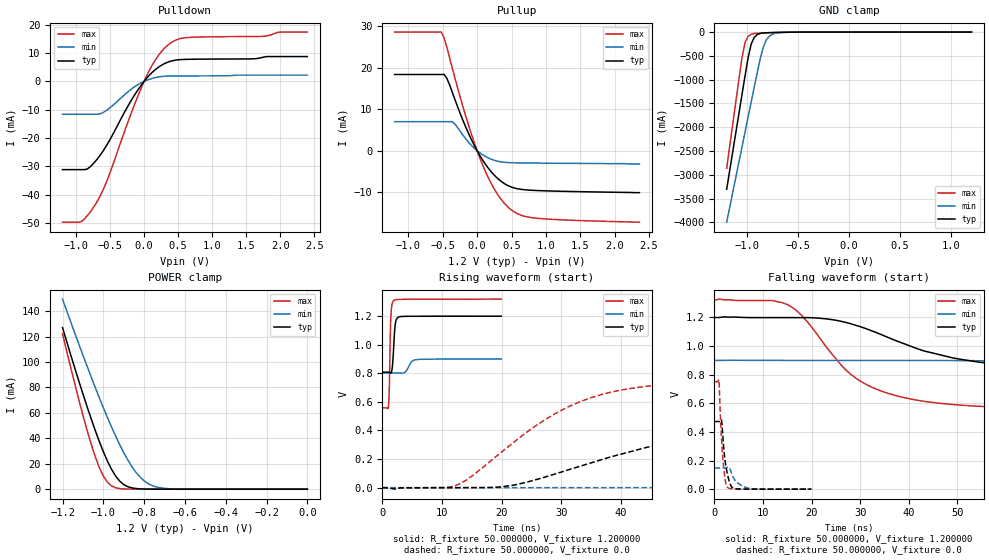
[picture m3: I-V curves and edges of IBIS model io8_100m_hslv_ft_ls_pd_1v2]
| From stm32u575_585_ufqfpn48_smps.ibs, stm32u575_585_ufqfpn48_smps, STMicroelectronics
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|   Model io8_100m_hslv_ft_ls_pd_1v2
[Model]  io8_100m_hslv_ft_ls_pd_1v2
Model_type I/O
Polarity   Non-Inverting
Enable   Active-Low
Vinl =   0.360000V
Vinh =   0.840000V
Vmeas =  0.600000V
Cref =   50.000000pF
Rref =   100.000000M
Vref =   0.0V
C_comp   3.030000pF   2.960800pF   3.078200pF
[Temperature Range]   25.000000   0.140000k   -40.000000
[Pullup Reference]   1.200000V   0.900000V   1.320000V
[Pulldown Reference]   0.0V   0.0V   0.0V
[POWER Clamp Reference]   1.200000V   0.900000V   1.320000V
[GND Clamp Reference]   0.0V   0.0V   0.0V
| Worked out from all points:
|   slope of the pulldown table from 0 to 0.18 V, typ, clamps not added: 40.7 ohm
|   slope of the pullup table from 0 to 0.18 V, typ, clamps not added: 39.5 ohm
|   GND clamp passes 1 mA (typ) near -0.51 V on its own axis
|   POWER clamp passes 1 mA (typ) near -0.86 V on its own axis
|   rising waveform, R_fixture 50.000000, V_fixture 1.200000: 20-80 % time 345ps typ, 818ps min, 226ps max; typ from 0.808 V to 1.2 V
|   rising waveform, R_fixture 50.000000, V_fixture 0.0: 20-80 % time 28.3ns typ, 68.2ns min, 16ns max; typ from 0 V to 0.472 V
|   falling waveform, R_fixture 50.000000, V_fixture 1.200000: 20-80 % time 23.6ns typ, 57ns min, 13.4ns max; typ from 1.2 V to 0.808 V
|   falling waveform, R_fixture 50.000000, V_fixture 0.0: 20-80 % time 1.03ns typ, 1.95ns min, 790ps max; typ from 0.472 V to 0 V
[Pulldown]
|Voltage   I(typ)   I(min)   I(max)
-1.2V     -31.16mA   -11.61mA   -49.71mA
-920mV    -31.16mA   -11.61mA   -49.48mA
-840mV    -31mA      -11.61mA   -47.54mA
-720mV    -28.33mA   -11.61mA   -43.58mA
-560mV    -22.95mA   -10.36mA   -35.89mA
-200mV    -7.146mA   -2.962mA   -11.89mA
0V        0A         -1.7pA     0A
160mV     4.047mA    1.297mA    7.361mA
360mV     6.87mA     1.868mA    13mA
640mV     7.765mA    1.921mA    15.46mA
1.76V     8.564mA    2.185mA    15.9mA
2.4V      8.742mA    2.185mA    17.38mA
[Pullup]
|Voltage   I(typ)   I(min)   I(max)
-1.2V     18.39mA    7.011mA    28.62mA
-520mV    18.39mA    7.011mA    28.62mA
-440mV    17.47mA    7.011mA    24.94mA
-360mV    14.06mA    7.011mA    19.88mA
-160mV    5.494mA    2.765mA    8.045mA
40mV      -1.16mA    -507.9uA   -1.774mA
240mV     -5.73mA    -2.255mA   -8.953mA
360mV     -7.518mA   -2.714mA   -11.96mA
480mV     -8.639mA   -2.875mA   -14.04mA
640mV     -9.31mA    -2.939mA   -15.55mA
880mV     -9.601mA   -2.983mA   -16.29mA
2.36V     -10.1mA    -3.2mA     -17.23mA
[GND_clamp]
|Voltage   I(typ)   I(min)   I(max)
-1.2V     -3.305A    -3.998A    -2.862A
-1.05V    -1.316A    -2.418A    -539.3mA
-1.02V    -921mA     -2.103A    -218.8mA
-990mV    -539.5mA   -1.788A    -87.45mA
-960mV    -252.2mA   -1.474A    -44.37mA
-930mV    -110.5mA   -1.16A     -30.33mA
-870mV    -28.04mA   -549.1mA   -21.1mA
-840mV    -18.44mA   -305.6mA   -18.29mA
-810mV    -13.92mA   -159.7mA   -15.75mA
-780mV    -11.24mA   -82.36mA   -13.39mA
-600mV    -2.986mA   -4.279mA   -3.072mA
1.2V      30.28uA    18.17uA    37.27uA
[POWER_clamp]
|Voltage   I(typ)   I(min)   I(max)
-1.2V     127mA      149.4mA    122.2mA
-1.12V    84.97mA    114mA      70.27mA
-1.06V    55.51mA    88.42mA    35.67mA
-1.02V    37.63mA    72.04mA    17.17mA
-1V       29.51mA    64.13mA    10.3mA
-960mV    15.69mA    48.99mA    2.571mA
-900mV    3.624mA    28.77mA    182.8uA
-840mV    490.7uA    13.24mA    11.35uA
-800mV    116.8uA    6.532mA    1.77uA
-740mV    13.2uA     1.723mA    109.1nA
-620mV    167.3nA    79.35uA    0A
0V        0A         17.84nA    0A
[Ramp]
| variable   typ   min   max
dV/dt_r  0.28337/28.24996n   88.70988m/68.15373n 0.45045/16.01538n
dV/dt_f  0.23483/23.46938n   58.00200m/56.89697n 0.45672/13.31776n
R_load = 50.000000
[Rising Waveform]
R_fixture= 50.000000
V_fixture= 1.200000
V_fixture_min= 0.900000
V_fixture_max= 1.320000
|time   V(typ)   V(min)   V(max)
0s        808mV      802.8mV    558.2mV
1.041ns   808.1mV    802.8mV    575.5mV
1.161ns   807.6mV    802.8mV    688.6mV
1.321ns   804.8mV    802.8mV    1.048V
1.441ns   802.6mV    802.8mV    1.207V
1.882ns   972.2mV    802.7mV    1.309V
2.202ns   1.154V     802.8mV    1.315V
2.843ns   1.195V     802.6mV    1.317V
5.726ns   1.199V     895.5mV    1.318V
19.94ns   1.199V     899.4mV    1.319V
[Rising Waveform]
R_fixture= 50.000000
V_fixture= 0.0
V_fixture_min= 0.0
V_fixture_max= 0.0
|time   V(typ)   V(min)   V(max)
0s        2.152nV    208.2nV    1.367nV
13.01ns   -87.29uV   -83.94uV   27.91mV
20.02ns   6.341mV    -72.32uV   250.3mV
27.03ns   71.13mV    -34.25uV   468.8mV
36.04ns   186.6mV    122.7uV    642.7mV
44.04ns   278.7mV    304.9uV    708.2mV
58.06ns   383.1mV    3.229mV    742.3mV
91.09ns   461.6mV    45.35mV    750.4mV
193.2ns   472.2mV    139.3mV    750.7mV
498.5ns   472.4mV    148mV      750.8mV
[Falling Waveform]
R_fixture= 50.000000
V_fixture= 1.200000
V_fixture_min= 0.900000
V_fixture_max= 1.320000
|time   V(typ)   V(min)   V(max)
0s        1.199V     899.4mV    1.319V
15.02ns   1.198V     899.3mV    1.29V
18.02ns   1.198V     899.1mV    1.211V
27.03ns   1.165V     899.1mV    832.7mV
34.03ns   1.084V     899.1mV    688.9mV
43.04ns   966.5mV    899mV      614.2mV
56.06ns   881.7mV    896.7mV    576.4mV
84.08ns   823.8mV    866.3mV    560.2mV
170.2ns   808.1mV    810.4mV    558.2mV
498.5ns   808mV      802.8mV    558.2mV
[Falling Waveform]
R_fixture= 50.000000
V_fixture= 0.0
V_fixture_min= 0.0
V_fixture_max= 0.0
|time   V(typ)   V(min)   V(max)
0s        472.4mV    148mV      750.8mV
920.9ps   472.8mV    148.1mV    762.3mV
1.441ns   484mV      148.1mV    361.2mV
1.682ns   392mV      148.2mV    236.7mV
2.202ns   195.8mV    148mV      66.69mV
2.683ns   103.7mV    152.5mV    12.79mV
3.684ns   9.798mV    96.8mV     1.508mV
4.805ns   1.729mV    43.64mV    259.3uV
6.927ns   39.01uV    7.412mV    118uV
19.94ns   2.152nV    208.2nV    1.367nV
